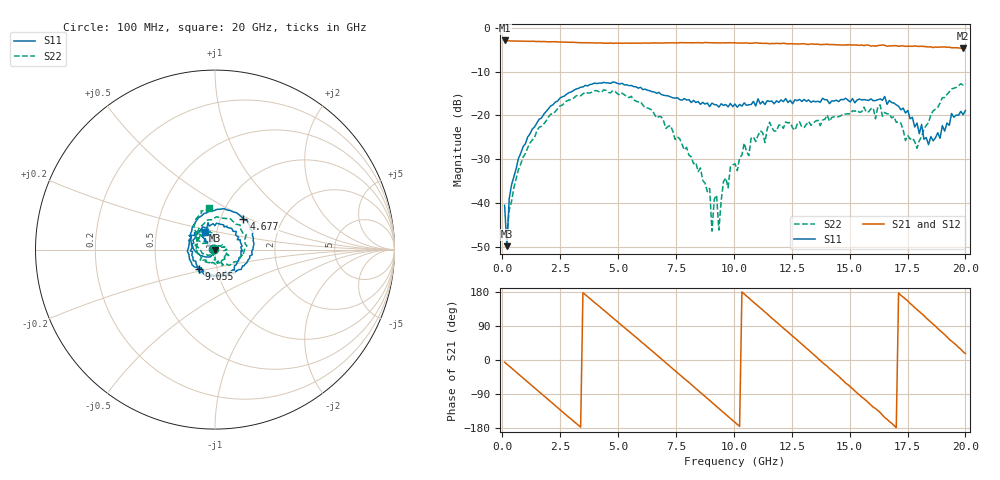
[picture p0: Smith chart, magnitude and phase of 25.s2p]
!Agilent Technologies,N5230C,MY49001569,A.09.33.09
!Agilent N5230C: A.09.33.09
!Date: Tuesday, July 28, 2015 14:51:03
!Correction: S11(Full 2 Port(1,2))
!S21(Full 2 Port(1,2))
!S12(Full 2 Port(1,2))
!S22(Full 2 Port(1,2))
!S2P File: Measurements: S11, S21, S12, S22:
# Hz S  dB  R 50
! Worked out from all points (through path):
!   201 points, 100 MHz to 20 GHz, reference 50 ohm
!   highest |S21| = -2.93 dB at 100 MHz (marker M1); lowest = -4.7 dB at 19.9 GHz (marker M2)
!   group delay of S21, straight-line fit = 147 ps
!   lowest |S11| = -49.8 dB at 199.5 MHz (marker M3), VSWR 1.01, Z = 49.8 - j0.284 ohm
!   |S11| at or under -10 dB: start of sweep to end of sweep
!   |S22| runs from -47.0 to -12.7 dB; largest |S21 - S12| = 0.023
!   S11 on the Smith chart (normalised r, x): 100 MHz: 0.98, +0.00; 4.677 GHz: 1.29, +0.46; 9.055 GHz: 0.82, -0.18; 20 GHz: 0.88, +0.18
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1e8  -40.45 164.6  -2.93 -5.7  -2.94 -5.9  -46.74 170.3
1.995e8  -49.75 -118.8  -2.99 -11.1  -3.03 -10.7  -47.05 -62.2
3.985e8  -35.81 -91.4  -3.04 -21.2  -3.04 -21.3  -39.59 -81.5
1.095e9  -24.94 -133.1  -3.11 -57.9  -3.11 -58.1  -27.37 -135.3
2.1895e9  -17.57 168.6  -3.22 -115.1  -3.23 -115.3  -19.63 162.0
3.483e9  -13.51 101.6  -3.45 177.6  -3.43 177.4  -15.10 91.1
4.677e9  -12.70 46.8  -3.50 116.3  -3.54 116.1  -14.86 30.6
6.7665e9  -14.76 -37.1  -3.48 8.3  -3.48 7.9  -20.25 -65.7
8.5575e9  -17.48 -108.0  -3.47 -85.7  -3.43 -86.4  -31.97 -118.2
8.9555e9  -17.99 -127.4  -3.45 -106.6  -3.49 -107.2  -36.61 -129.8
9.055e9  -17.18 -130.2  -3.45 -112.1  -3.46 -112.5  -46.33 166.1
9.1545e9  -17.53 -139.3  -3.47 -117.4  -3.49 -117.8  -39.05 149.6
9.3535e9  -18.10 -148.9  -3.50 -127.6  -3.49 -128.4  -46.09 179.5
1.005e10  -17.39 168.5  -3.45 -164.6  -3.52 -165.2  -30.99 62.7
1.1841e10  -16.67 63.0  -3.59 99.8  -3.66 99.6  -23.54 -38.9
1.3433e10  -16.70 -26.1  -3.77 15.2  -3.80 13.9  -21.76 -117.9
1.5224e10  -17.12 -134.4  -3.94 -81.5  -4.01 -81.5  -19.06 164.4
1.67165e10  -16.60 140.9  -4.17 -162.3  -4.08 -163.3  -19.58 101.1
1.79105e10  -21.72 103.0  -4.25 133.3  -4.29 132.7  -27.46 131.8
1.8408e10  -26.64 131.1  -4.41 105.3  -4.32 104.6  -21.64 150.3
1.99005e10  -19.84 121.5  -4.74 22.0  -4.62 21.6  -13.08 103.9
2e10  -18.88 119.2  -4.71 16.9  -4.65 16.4  -12.70 98.8
